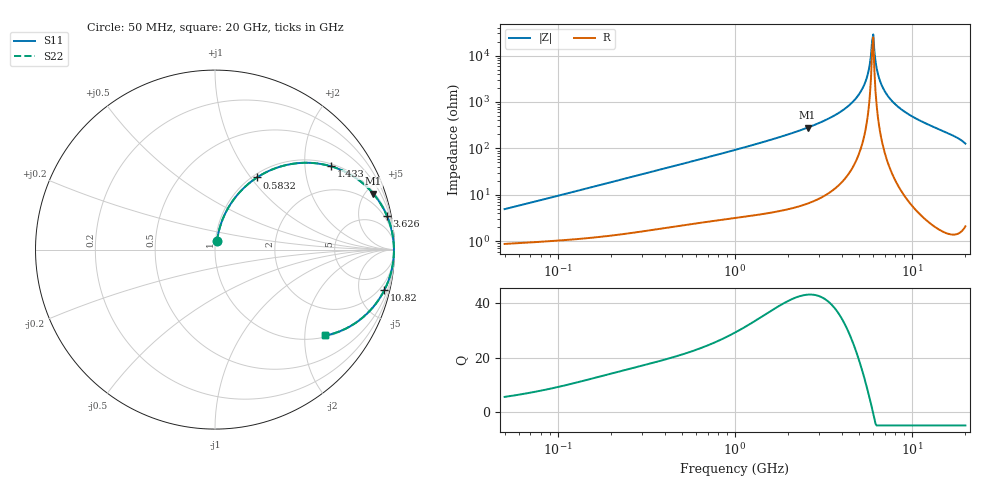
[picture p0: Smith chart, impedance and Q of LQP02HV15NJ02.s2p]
!Murata Part Number: LQP02HV15NJ02
!These Parameters are Measured in Series Mode Connection
!  o--[Z]--o
!Port1  Port2
!  o-------o
!Freq. Start=50[MHz] Stop=20[GHz], 401[Steps]
# Hz S RI R 50
!Freq.(Hz) S11(Real) S11(Imag) S21(Real) S21(Imag) S12(Real) S12(Imag) S22(Real) S22(Imag)
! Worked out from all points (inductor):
!   401 points, 50 MHz to 20 GHz, reference 50 ohm
!   read as one part in series: L = 15.3 nH near 51.52 MHz
!   highest Q = 43.3 at 2.569 GHz (marker M1), where L = 17.4 nH
!   self-resonance near 5.944 GHz
!   S11 on the Smith chart (normalised r, x): 50 MHz: 1.02, +0.10; 583.2 MHz: 1.05, +1.07; 1.433 GHz: 1.08, +2.73; 3.626 GHz: 1, +10; 10.82 GHz: 1.08, -8.33; 20 GHz: 1.04, -2.54
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5e7  0.011 0.0475  0.989 -0.0475  0.989 -0.0475  0.011 0.0475
1.364002e8  0.027 0.1237  0.973 -0.1237  0.973 -0.1237  0.027 0.1237
3.721004e8  0.1188 0.298  0.8812 -0.298  0.8812 -0.298  0.1188 0.298
5.831961e8  0.234 0.4018  0.766 -0.4018  0.766 -0.4018  0.234 0.4018
1e9  0.464 0.4819  0.536 -0.4819  0.536 -0.4819  0.464 0.4819
1.432596e9  0.6463 0.4642  0.3537 -0.4642  0.3537 -0.4642  0.6463 0.4642
2.569357e9  0.8818 0.3115  0.1182 -0.3115  0.1182 -0.3115  0.8818 0.3115
2.728004e9  0.8984 0.2907  0.1016 -0.2907  0.1016 -0.2907  0.8984 0.2907
3.626126e9  0.9582 0.1877  0.0418 -0.1877  0.0418 -0.1877  0.9582 0.1877
4.472136e9  0.9837 0.1099  0.0163 -0.1099  0.0163 -0.1099  0.9837 0.1099
5.117541e9  0.9929 0.0597  0.00707 -0.0597  0.00707 -0.0597  0.9929 0.0597
5.515528e9  0.9957 0.0318  0.00428 -0.0318  0.00428 -0.0318  0.9957 0.0318
5.683258e9  0.9964 0.0207  0.00361 -0.0207  0.00361 -0.0207  0.9964 0.0207
5.856089e9  0.9968 0.00947  0.00319 -0.00947  0.00319 -0.00947  0.9968 0.00947
6.034176e9  0.997 -0.00173  0.00304 0.00173  0.00304 0.00173  0.997 -0.00173
6.125241e9  0.9969 -0.00733  0.00305 0.00733  0.00305 0.00733  0.9969 -0.00733
6.406762e9  0.9965 -0.0242  0.00349 0.0242  0.00349 0.0242  0.9965 -0.0242
6.601595e9  0.9959 -0.0354  0.00411 0.0354  0.00411 0.0354  0.9959 -0.0354
7.442007e9  0.9908 -0.0807  0.00923 0.0807  0.00923 0.0807  0.9908 -0.0807
1.082228e10  0.9435 -0.226  0.0565 0.226  0.0565 0.226  0.9435 -0.226
1.597544e10  0.8163 -0.3838  0.1837 0.3838  0.1837 0.3838  0.8163 -0.3838
2e10  0.6151 -0.4784  0.3849 0.4784  0.3849 0.4784  0.6151 -0.4784
